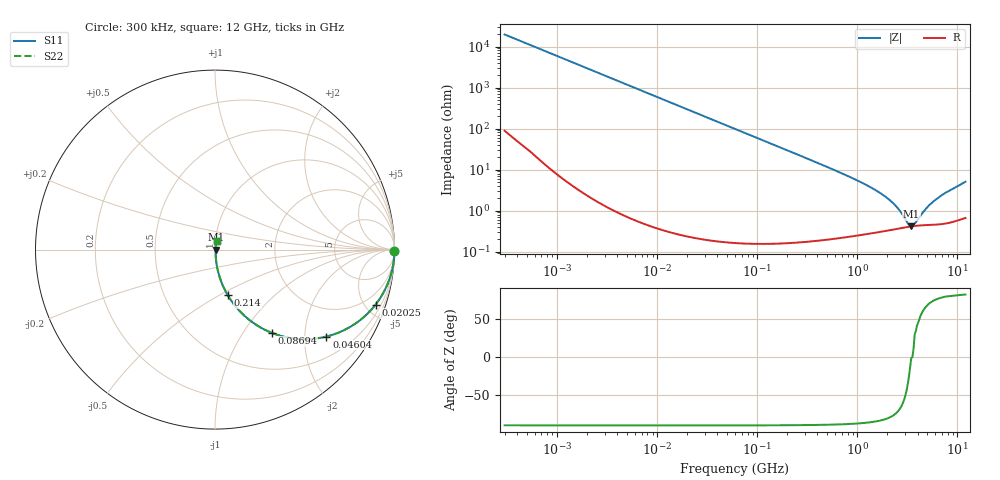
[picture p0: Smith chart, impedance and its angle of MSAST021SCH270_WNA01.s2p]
! MSAST021SCH270_WNA01  S-PARAMETER MODEL  ( General Type )
! Model Generated by TAIYO YUDEN Corporation (http://www.ty-top.com)
! Version 2.0
! TAIYO YUDEN Control No. 181101
! Copyright(c) 2016 TAIYO YUDEN CO.,LTD. All Rights Reserved.
! Product Description (link to TY-COMPAS)
! https://ds.yuden.co.jp/TYCOMPAS/or/detail?pn=MSAST021SCH270JWNA01&u=M
! Products Name : Multilayer Ceramic Capacitors
! Characteristics :
!  Capacitance : 27 pF , Rated Voltage : 25V , TCC : CH / C0H
!  Case Size : 0.25 x 0.125 / 0.0098 x 0.0049 [mm/inch] , Thickness : 0.125 / 0.0049 [mm/inch]
!  (Conditions: Temperature = 25 degC , DC Bias Current/Voltage = 0A / 0V)
! External Node Assignments :
!  1  o---| |---o  2
! GND o---------o GND
! Frequency Range : 0.3MHz  -  12000MHz  [ 401 STEP ]
# MHz S RI R 50
! Freq[MHz].  S11 Real  S11 Imag  S21 Real  S21 Imag  S12 Real  S12 Imag  S22 Real  S22 Imag
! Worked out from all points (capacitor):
!   401 points, 300 kHz to 12 GHz, reference 50 ohm
!   read as one part in series: C = 27 pF near 316.3 kHz
!   lowest |Z| = 410 mohm at 3.455 GHz (marker M1)
!   series resonance near 3.537 GHz, so ESL is about 75 pH
!   S11 on the Smith chart (normalised r, x): 300 kHz: open; 20.25 MHz: 1.00, -5.82; 46.04 MHz: 1.00, -2.56; 86.94 MHz: 1.00, -1.36; 214 MHz: 1.00, -0.55; 12 GHz: 1.01, +0.10
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0.3  1 -0.00509  4.87e-05 0.00509  4.87e-05 0.00509  1 -0.00509
1.769972  0.9991 -0.03  0.000926 0.03  0.000926 0.03  0.9991 -0.03
4.84353  0.9932 -0.0816  0.00675 0.0816  0.00675 0.0816  0.9932 -0.0816
10.44266  0.9695 -0.1717  0.0305 0.1717  0.0305 0.1717  0.9695 -0.1717
20.2507  0.8942 -0.3071  0.1058 0.3071  0.1058 0.3071  0.8942 -0.3071
30.13126  0.7926 -0.405  0.2074 0.405  0.2074 0.405  0.7926 -0.405
46.03623  0.6209 -0.4845  0.3791 0.4845  0.3791 0.4845  0.6209 -0.4845
60  0.491 -0.4991  0.509 0.4991  0.509 0.4991  0.491 -0.4991
86.94074  0.315 -0.4634  0.685 0.4634  0.685 0.4634  0.315 -0.4634
132.8329  0.165 -0.3694  0.835 0.3694  0.835 0.3694  0.165 -0.3694
213.9924  0.0713 -0.2544  0.9287 0.2544  0.9287 0.2544  0.0713 -0.2544
353.9943  0.0281 -0.1599  0.9719 0.1599  0.9719 0.1599  0.0281 -0.1599
1135.593  0.00469 -0.046  0.9953 0.046  0.9953 0.046  0.00469 -0.046
2088.533  0.0036 -0.0179  0.9964 0.0179  0.9964 0.0179  0.0036 -0.0179
2514.07  0.0037 -0.011  0.9963 0.011  0.9963 0.011  0.0037 -0.011
3190.978  0.00398 -0.0028  0.996 0.0028  0.996 0.0028  0.00398 -0.0028
3454.93  0.00409 -0.000108  0.9959 0.000108  0.9959 0.000108  0.00409 -0.000108
3740.715  0.00419 0.00242  0.9958 -0.00242  0.9958 -0.00242  0.00419 0.00242
4747.894  0.00447 0.00939  0.9955 -0.00939  0.9955 -0.00939  0.00447 0.00939
5868.704  0.00477 0.0167  0.9952 -0.0167  0.9952 -0.0167  0.00477 0.0167
7448.838  0.00541 0.0256  0.9946 -0.0256  0.9946 -0.0256  0.00541 0.0256
12000  0.00897 0.0491  0.991 -0.0491  0.991 -0.0491  0.00897 0.0491
